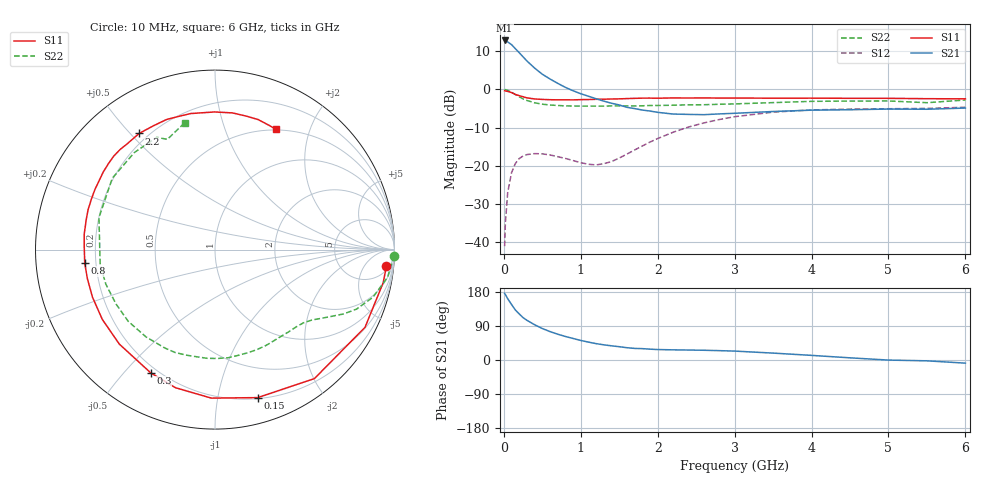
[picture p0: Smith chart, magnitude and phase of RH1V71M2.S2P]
! SIEMENS Small Signal Semiconductors
! BFR106
! Si NPN RF Bipolar Junction Transistor in SOT23
! VCE = 1.75 V  IC = 1.2 mA
! Common Emitter S-Parameters:  August  1996
# GHz  S  MA  R  50
!  f  S11  S21  S12  S22
! GHz  MAG  ANG  MAG  ANG  MAG  ANG  MAG  ANG
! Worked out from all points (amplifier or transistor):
!   36 points, 10 MHz to 6 GHz, reference 50 ohm
!   highest |S21| = 12.8 dB at 10 MHz (marker M1)
!   |S21| within 3 dB of that: start of sweep to 190.1 MHz
!   unconditionally stable (mu >= 1): 839.5 MHz to end of sweep
!   at 250 MHz: K = 0.28, MSG = 13.0 dB, |S12| = -17.5 dB
!   at 1.4 GHz: K = 1.47, MAG = 3.6 dB, |S12| = -18.9 dB
!   at 6 GHz: K = 1.02, MAG = -1.0 dB, |S12| = -4.7 dB
!   S11 on the Smith chart (normalised r, x): 10 MHz: 7, -17; 150 MHz: 0.21, -1.31; 300 MHz: 0.17, -0.59; 800 MHz: 0.16, -0.05; 2.2 GHz: 0.16, +0.53; 6 GHz: 0.49, +1.52
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0.01  0.9593 -5.6  4.38 175.8  0.0088 87.5  0.9992 -2.0
0.02  0.9552 -11.1  4.368 172.8  0.0178 84.9  0.9906 -3.7
0.05  0.9413 -27.4  4.187 161.7  0.0443 74.4  0.9736 -9.1
0.1  0.9074 -52.4  3.862 146.5  0.0808 61.1  0.9191 -16.8
0.15  0.8583 -73.9  3.414 131.9  0.107 49.1  0.8556 -22.8
0.2  0.8278 -91.4  3.028 121.6  0.1239 40.8  0.8007 -26.6
0.25  0.8004 -106.0  2.672 111.8  0.1339 33.7  0.7499 -29.7
0.3  0.7743 -117.6  2.359 104.8  0.1397 28.8  0.7156 -32.1
0.4  0.7492 -135.3  1.902 93.0  0.1439 21.3  0.6674 -36.0
0.5  0.7386 -148.2  1.581 83.1  0.1428 16.7  0.6398 -39.6
0.6  0.7323 -158.7  1.368 75.0  0.1382 14.3  0.6242 -43.7
0.8  0.7297 -174.1  1.063 62.1  0.1245 13.6  0.6077 -52.6
1.1  0.7363 167.3  0.813 47.2  0.1043 25.7  0.6041 -67.3
1.3  0.7439 157.8  0.701 40.0  0.1062 41.3  0.6033 -77.8
1.6  0.7581 145.2  0.582 32.4  0.1418 59.6  0.6073 -94.1
2.2  0.7728 123.1  0.475 26.8  0.2742 61.9  0.62 -128.3
2.8  0.7693 105.2  0.477 24.7  0.4025 48.4  0.6379 -162.4
3.5  0.7669 90.2  0.513 18.2  0.5032 31.2  0.6707 164.6
4.5  0.7638 76.8  0.541 5.7  0.5513 11.0  0.7031 129.8
5  0.7633 71.6  0.552 -0.2  0.5576 3.7  0.7048 117.4
5.5  0.7551 66.6  0.549 -2.2  0.5629 0.4  0.6691 113.4
6  0.7513 63.0  0.569 -8.3  0.5835 -7.0  0.7258 103.5
